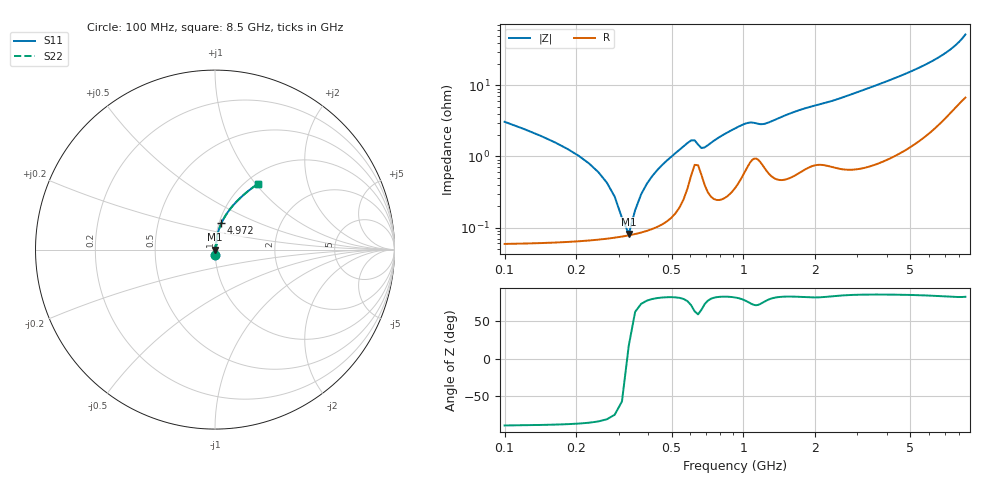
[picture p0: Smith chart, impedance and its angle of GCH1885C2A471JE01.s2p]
!Murata Part Number: GCH1885C2A471JE01
!These Parameters are Measured in Series Mode Connection
!Data Generated on Jun 19, 2026
!  o--ll--o
!Port1  Port2
!  o------o
!Operation Temp=25[degC], DC Bias Voltage=0[V]
!Freq. Start=100[MHz] Stop=9[GHz] 401[Steps]
# Hz S RI R 50
!Freq.(Hz) S11(Real) S11(Imag) S21(Real) S21(Imag) S12(Real) S12(Imag) S22(Real) S22(Imag)
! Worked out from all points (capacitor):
!   401 points, 100 MHz to 8.5 GHz, reference 50 ohm
!   read as one part in series: C = 468 pF near 142 MHz
!   lowest |Z| = 81.3 mohm at 331 MHz (marker M1)
!   series resonance near 327.3 MHz, so ESL is about 510 pH
!   S11 on the Smith chart (normalised r, x): 100 MHz: 1.00, -0.06; 4.972 GHz: 1.03, +0.31; 8.5 GHz: 1.13, +1.03
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1e8  0.00153 -0.0307  0.9985 0.0307  0.9985 0.0307  0.00153 -0.0307
1.42e8  0.000981 -0.0194  0.999 0.0194  0.999 0.0194  0.000981 -0.0194
2.05e8  0.000744 -0.0101  0.9993 0.0101  0.9993 0.0101  0.000744 -0.0101
2.47e8  0.000711 -0.00597  0.9993 0.00597  0.9993 0.00597  0.000711 -0.00597
2.89e8  0.000726 -0.00262  0.9993 0.00262  0.9993 0.00262  0.000726 -0.00262
3.1e8  0.000747 -0.00114  0.9993 0.00114  0.9993 0.00114  0.000747 -0.00114
3.31e8  0.000776 0.000242  0.9992 -0.000242  0.9992 -0.000242  0.000776 0.000242
3.52e8  0.000813 0.00155  0.9992 -0.00155  0.9992 -0.00155  0.000813 0.00155
3.94e8  0.000913 0.00402  0.9991 -0.00402  0.9991 -0.00402  0.000913 0.00402
4.36e8  0.00106 0.00636  0.9989 -0.00636  0.9989 -0.00636  0.00106 0.00636
4.99e8  0.00147 0.00983  0.9985 -0.00983  0.9985 -0.00983  0.00147 0.00983
5.83e8  0.00375 0.015  0.9962 -0.015  0.9962 -0.015  0.00375 0.015
7.09e8  0.00334 0.0139  0.9967 -0.0139  0.9967 -0.0139  0.00334 0.0139
1.024e9  0.00724 0.028  0.9928 -0.028  0.9928 -0.028  0.00724 0.028
1.234e9  0.00739 0.0278  0.9926 -0.0278  0.9926 -0.0278  0.00739 0.0278
1.507e9  0.00615 0.0376  0.9938 -0.0376  0.9938 -0.0376  0.00615 0.0376
2.914e9  0.0123 0.0759  0.9877 -0.0759  0.9877 -0.0759  0.0123 0.0759
4.3e9  0.0252 0.1216  0.9748 -0.1216  0.9748 -0.1216  0.0252 0.1216
4.972e9  0.0355 0.1468  0.9645 -0.1468  0.9645 -0.1468  0.0355 0.1468
5.707e9  0.0516 0.1779  0.9484 -0.1779  0.9484 -0.1779  0.0516 0.1779
7.114e9  0.1066 0.2528  0.8934 -0.2528  0.8934 -0.2528  0.1066 0.2528
8.5e9  0.241 0.3675  0.759 -0.3675  0.759 -0.3675  0.241 0.3675
